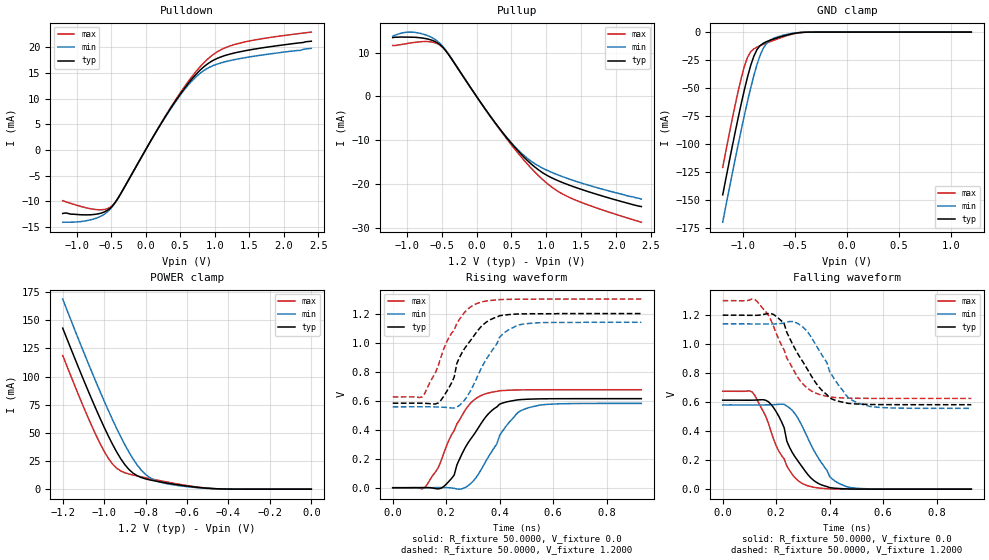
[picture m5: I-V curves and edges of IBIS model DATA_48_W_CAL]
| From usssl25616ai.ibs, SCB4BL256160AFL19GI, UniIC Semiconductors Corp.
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|   Model DATA_48_W_CAL
[Model]  DATA_48_W_CAL
Model_type I/O
Polarity   Non-Inverting
Enable   Active-High
Vinl =   0.3800V
Vinh =   0.8200V
Vmeas =  0.6000V
Cref =   5.0000pF
Rref =   50.0000
Vref =   0.6000V
C_comp   1.7430pF   1.7110pF   1.7640pF
[Temperature Range]   25.0000   85.0000   -40.0000
[Voltage Range]   1.2000V   1.1400V   1.3000V
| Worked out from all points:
|   slope of the pulldown table from 0 to 0.18 V, typ, clamps not added: 43.4 ohm
|   slope of the pullup table from 0 to 0.18 V, typ, clamps not added: 43.8 ohm
|   GND clamp passes 1 mA (typ) near -0.50 V on its own axis
|   POWER clamp passes 1 mA (typ) near -0.51 V on its own axis
|   rising waveform, R_fixture 50.0000, V_fixture 0.0: 20-80 % time 114ps typ, 115ps min, 104ps max; typ from 0 V to 0.614 V
|   rising waveform, R_fixture 50.0000, V_fixture 1.2000: 20-80 % time 100ps typ, 104ps min, 102ps max; typ from 0.582 V to 1.2 V
|   falling waveform, R_fixture 50.0000, V_fixture 0.0: 20-80 % time 96.3ps typ, 105ps min, 97.6ps max; typ from 0.614 V to 0 V
|   falling waveform, R_fixture 50.0000, V_fixture 1.2000: 20-80 % time 118ps typ, 113ps min, 105ps max; typ from 1.2 V to 0.582 V
[Pulldown]
|Voltage   I(typ)   I(min)   I(max)
-1.2V     -12.4mA    -14.1mA    -9.9mA
-720mV    -12.55mA   -13.35mA   -11.64mA
-600mV    -12.12mA   -12.58mA   -11.63mA
-480mV    -10.93mA   -11.05mA   -10.84mA
-360mV    -8.541mA   -8.522mA   -8.575mA
80mV      1.872mA    1.857mA    1.895mA
360mV     8.045mA    7.937mA    8.192mA
640mV     13.34mA    12.99mA    13.74mA
840mV     16.17mA    15.45mA    16.94mA
1.04V     17.86mA    16.75mA    19.15mA
1.28V     18.88mA    17.59mA    20.52mA
2.4V      21.2mA     19.8mA     22.98mA
[Pullup]
|Voltage   I(typ)   I(min)   I(max)
-1.2V     13.4mA     13.7mA     11.6mA
-1V       13.52mA    14.63mA    12.03mA
-800mV    13.36mA    14.35mA    12.46mA
-600mV    12.55mA    13.05mA    12.26mA
-480mV    11.14mA    11.34mA    11.15mA
120mV     -2.766mA   -2.805mA   -2.797mA
360mV     -7.948mA   -7.962mA   -8.132mA
640mV     -13.19mA   -12.9mA    -13.79mA
840mV     -16.16mA   -15.38mA   -17.31mA
1.08V     -18.58mA   -17.33mA   -20.7mA
1.32V     -20.18mA   -18.79mA   -22.95mA
2.36V     -25.1mA    -23.4mA    -28.67mA
[GND_clamp]
|Voltage   I(typ)   I(min)   I(max)
-1.2V     -145.3mA   -169.7mA   -120.8mA
-1.11V    -103.1mA   -127.3mA   -78.51mA
-1.05V    -76.2mA    -100.1mA   -52.43mA
-990mV    -51.2mA    -74mA      -30.39mA
-960mV    -39.9mA    -61.63mA   -22.48mA
-900mV    -21.67mA   -39mA      -15mA
-870mV    -15.78mA   -29.25mA   -13.45mA
-810mV    -10.04mA   -14.72mA   -11.07mA
-750mV    -7.557mA   -7.71mA    -8.865mA
-600mV    -3.111mA   -2.463mA   -3.804mA
-420mV    -215.4uA   -156.1uA   -235uA
1.2V      1.597nA    5.589nA    1.463nA
[POWER_clamp]
|Voltage   I(typ)   I(min)   I(max)
-1.2V     143mA      168.8mA    118.7mA
-1.06V    79.88mA    104.3mA    56.26mA
-1.02V    63.08mA    86.79mA    40.63mA
-980mV    47.32mA    69.97mA    27.48mA
-940mV    33.2mA     54.05mA    18.67mA
-880mV    17.43mA    32.78mA    13.45mA
-840mV    11.87mA    21.34mA    11.69mA
-800mV    9.133mA    13.1mA     10.12mA
-720mV    6.135mA    5.731mA    7.166mA
-560mV    1.838mA    1.456mA    2.161mA
-420mV    156.9uA    132.7uA    153uA
0V        1.597nA    1.927nA    2.16nA
[Ramp]
| variable   typ   min   max
dV/dt_r  0.3682/0.1099n   0.3486/0.1160n   0.4051/0.1060n
dV/dt_f  0.3705/0.1101n   0.3496/0.1150n   0.4045/0.1066n
R_load = 50.0000
[Rising Waveform]
R_fixture= 50.0000
V_fixture= 0.0
V_fixture_min= 0.0
V_fixture_max= 0.0
|time   V(typ)   V(min)   V(max)
0s        0V         0V         0V
120ps     1.127mV    198.7uV    896.5uV
170ps     -8.205mV   1.015mV    136.8mV
190ps     7.022mV    1.412mV    232.2mV
230ps     87.34mV    -4.218mV   394.5mV
270ps     272.4mV    206.3uV    531.1mV
340ps     468.3mV    154.8mV    642.4mV
420ps     588.3mV    414mV      670.5mV
490ps     608.5mV    539.2mV    674.4mV
930ps     613.7mV    581mV      675.2mV
[Rising Waveform]
R_fixture= 50.0000
V_fixture= 1.2000
V_fixture_min= 1.1400
V_fixture_max= 1.3000
|time   V(typ)   V(min)   V(max)
0s        582.5mV    557.4mV    625.9mV
110ps     582.1mV    557.7mV    625.6mV
170ps     583.7mV    556.2mV    838.9mV
220ps     721.7mV    549.4mV    1.064V
250ps     898.1mV    567.5mV    1.161V
280ps     987.7mV    633.2mV    1.229V
320ps     1.087V     778.9mV    1.273V
400ps     1.185V     1.038V     1.296V
470ps     1.197V     1.121V     1.299V
930ps     1.2V       1.14V      1.3V
[Falling Waveform]
R_fixture= 50.0000
V_fixture= 0.0
V_fixture_min= 0.0
V_fixture_max= 0.0
|time   V(typ)   V(min)   V(max)
0s        613.7mV    581mV      675.2mV
110ps     613.6mV    580.7mV    670.8mV
170ps     603.9mV    581.4mV    459.5mV
220ps     465mV      585.9mV    232.2mV
250ps     288.7mV    560mV      129.5mV
310ps     120.9mV    384.9mV    28.64mV
350ps     47.7mV     238.4mV    10.21mV
400ps     10.85mV    86.97mV    2.161mV
460ps     2.161mV    19.68mV    403.9uV
930ps     0V         0V         0V
[Falling Waveform]
R_fixture= 50.0000
V_fixture= 1.2000
V_fixture_min= 1.1400
V_fixture_max= 1.3000
|time   V(typ)   V(min)   V(max)
0s        1.2V       1.14V      1.3V
120ps     1.199V     1.139V     1.308V
170ps     1.211V     1.139V     1.203V
200ps     1.192V     1.14V      1.076V
230ps     1.14V      1.146V     958.5mV
280ps     936.5mV    1.143V     774mV
350ps     728.4mV    990.1mV    661.1mV
430ps     608.1mV    725.8mV    631.1mV
500ps     587.6mV    598.8mV    626.8mV
930ps     582.5mV    557.4mV    625.9mV
